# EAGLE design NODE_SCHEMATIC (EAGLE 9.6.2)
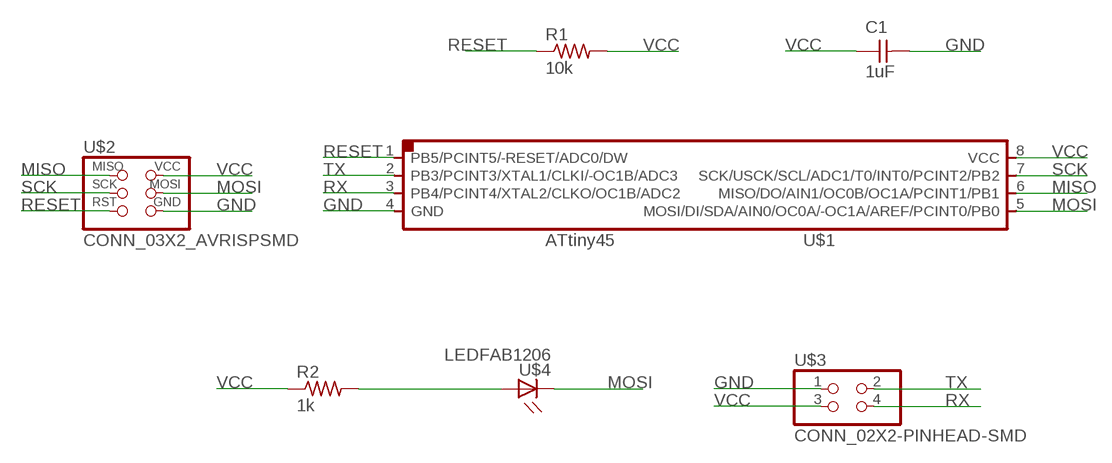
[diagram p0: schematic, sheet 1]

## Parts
C1  1uF  CAP_UNPOLARIZEDFAB  [C1206FAB]
R1  10k  R1206FAB  [R1206FAB]
R2  1k  R1206FAB  [R1206FAB]
U$1  UC_ATTINY45SI  [SOIC8]
U$2  CONN_03X2_AVRISPSMD  [2X03SMD]
U$3  CONN_02X2-PINHEAD-SMD  [2X02SMD]
U$4  LEDFAB1206  [LED1206FAB]

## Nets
GND: C1.2 U$1.4(GND) U$2.6(GND) U$3.1
MISO: U$1.6(MISO/DO/AIN1/OC0B/OC1A/PCINT1/PB1) U$2.1(MISO)
MOSI: U$1.5(MOSI/DI/SDA/AIN0/OC0A/-OC1A/AREF/PCINT0/PB0) U$2.4(MOSI) U$4.2(C)
N$1: R2.2 U$4.1(A)
RESET: R1.1 U$1.1(PB5/PCINT5/-RESET/ADC0/DW) U$2.5(RST)
RX: U$1.3(PB4/PCINT4/XTAL2/CLKO/OC1B/ADC2) U$3.4
SCK: U$1.7(SCK/USCK/SCL/ADC1/T0/INT0/PCINT2/PB2) U$2.3(SCK)
TX: U$1.2(PB3/PCINT3/XTAL1/CLKI/-OC1B/ADC3) U$3.2
VCC: C1.1 R1.2 R2.1 U$1.8(VCC) U$2.2(VCC) U$3.3

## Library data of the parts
C1 = fab:CAP_UNPOLARIZED
R1 R2 = fab:R: Resistor (US Symbol)
U$1 = fab:UC_ATTINY45
U$2 = fab:CONN_03X2_AVRISP
U$3 = fab:CONN_02X2-PINHEAD-SMD
U$4 = fab:LED: LED

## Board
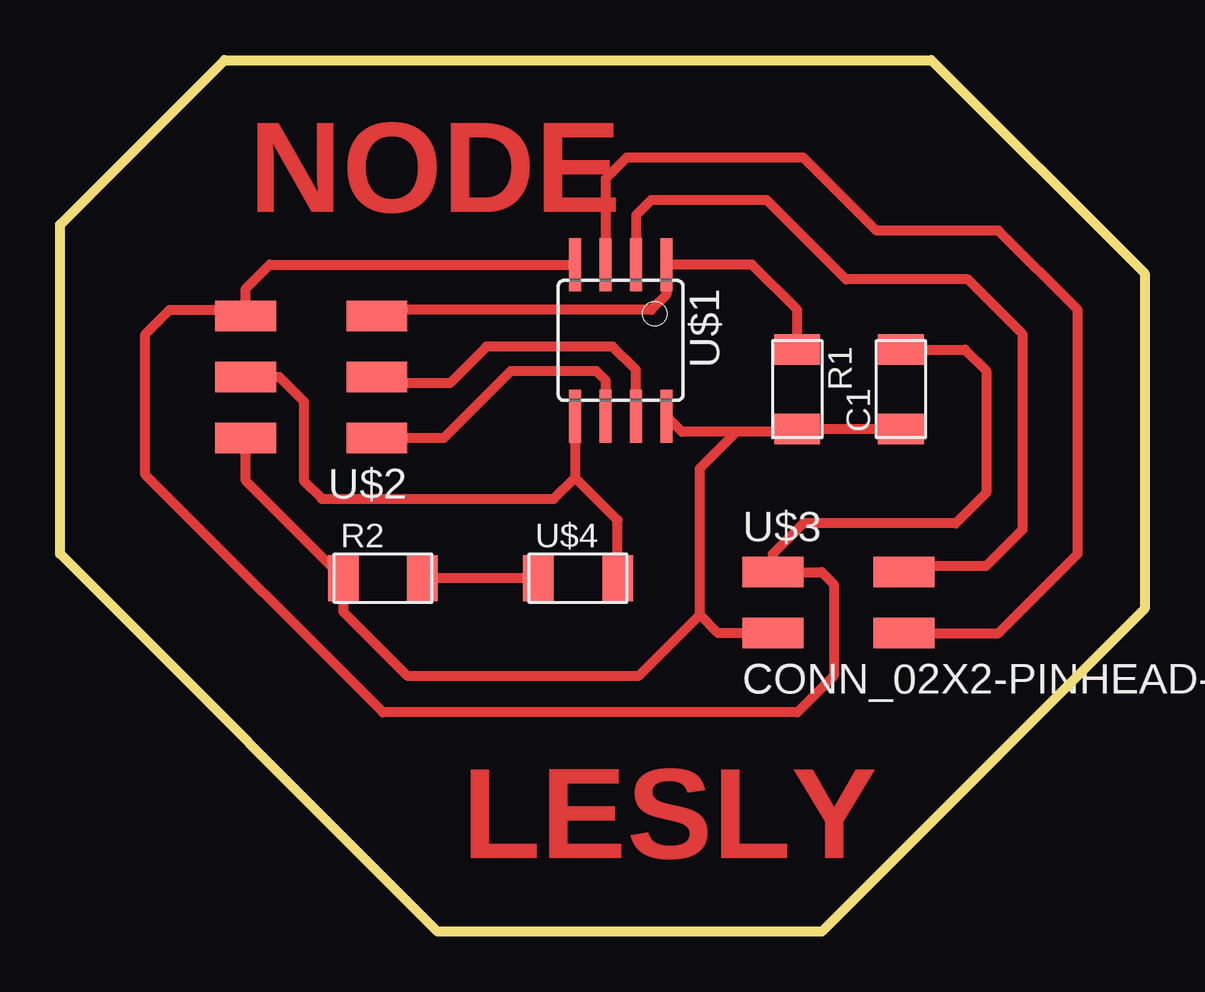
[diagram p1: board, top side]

Size 45.21 x 36.32 mm. Coordinates in mm from the lower left corner, seen from the top.
Outline: 0,29.46 6.86,36.32 36.32,36.32 45.21,27.43 45.21,13.46 31.75,0 15.75,0 0,15.75 0,17.78 0,18.03 0,29.46
Copper layers (1*16): Top 0.035mm / dielectric 1.5mm / Bottom 0.035mm
Design rules "fab": minimum track width 10mil, minimum drill 32mil, track to track 16mil, track to pad 16mil, pad to pad 16mil, via to via 16mil, smd to smd 6mil, copper to edge 16mil, drill to drill 16mil, minimum pad ring 10mil, minimum via ring 8mil, stop-mask expansion 4mil, vias tented up to drill 0mil, thermal gap 16mil

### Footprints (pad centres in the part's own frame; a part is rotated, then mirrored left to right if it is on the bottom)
C1206FAB = smd 1.27 x 1.905: 1 -1.651,0; 2 1.651,0
R1206FAB = smd 1.27 x 1.905: 1 -1.651,0; 2 1.651,0
SOIC8 = smd 0.5 x 2.2: 1 -1.905,-3.154; 2 -0.645,-3.154; 3 0.625,-3.154; 4 1.895,-3.154; 5 1.905,3.154; 6 0.635,3.154; 7 -0.635,3.154; 8 -1.905,3.154
2X03SMD = smd 2.54 x 1.27: 1 -2.54,2.54; 2 2.92,2.54; 3 -2.54,0; 4 2.92,0; 5 -2.54,-2.54; 6 2.92,-2.54
2X02SMD = smd 2.54 x 1.27: 1 -2.54,1.27; 2 2.92,1.27; 3 -2.54,-1.27; 4 2.92,-1.27
LED1206FAB = smd 1.27 x 1.905: 1 -1.651,0; 2 1.651,0

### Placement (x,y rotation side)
C1  35.05,22.61 90 top
R1  30.73,22.61 270 top
R2  13.46,14.73 0 top
U$1  23.37,24.64 180 top
U$2  10.67,23.11 180 top
U$3  32.26,13.72 0 top
U$4  21.59,14.73 0 top

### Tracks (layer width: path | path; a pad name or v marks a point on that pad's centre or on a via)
GND
  Top 0.406: C1.2 37.72,24.26 38.61,23.37 38.61,18.29 37.34,17.02 30.99,17.02 29.72,15.75 U$3.1 31.75,14.99 32.26,14.48 32.26,10.67 30.73,9.14 13.46,9.14 3.56,19.05 3.56,24.89 4.57,25.91 7.49,25.91 U$2.6 7.75,26.8 8.74,27.79 U$1.4
MISO
  Top 0.406: U$2.1 16,20.57 18.8,23.37 22.35,23.37 22.73,22.99 U$1.6
MOSI
  Top 0.406: U$4.2 23.24,17.14 21.46,18.92 | U$1.5 21.46,18.92 | U$2.4 9.14,23.11 10.16,22.1 10.16,18.8 10.92,18.03 20.57,18.03 21.46,18.92
N$1
  Top 0.406: U$4.1 R2.2
RESET
  Top 0.406: R1.1 30.73,25.91 28.85,27.79 U$1.1 25.27,26.54 24.64,25.91 13.46,25.91 U$2.5
RX
  Top 0.406: U$3.4 39.12,12.45 42.42,15.75 42.42,25.91 39.12,29.21 34.04,29.21 30.99,32.26 23.62,32.26 22.74,31.38 U$1.3
SCK
  Top 0.406: U$1.7 24,23.42 23.04,24.38 17.78,24.38 16.26,22.86 13.46,22.86 U$2.3
TX
  Top 0.406: U$3.2 35.43,15.24 38.61,15.24 40.13,16.76 40.13,24.89 37.85,27.18 32.77,27.18 29.46,30.48 24.64,30.48 24.01,29.86 U$1.2
VCC
  Top 0.406: C1.1 R1.2 30.61,20.83 28.19,20.83 | U$1.8 25.93,20.83 28.19,20.83 | U$2.2 7.75,18.8 R2.1 11.81,13.34 14.48,10.67 24.13,10.67 26.67,13.21 | 26.67,13.21 26.67,16.76 26.67,16.89 26.67,19.3 28.19,20.83 | U$3.3 27.43,12.45 26.67,13.21

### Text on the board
Top: NODE | LESLY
